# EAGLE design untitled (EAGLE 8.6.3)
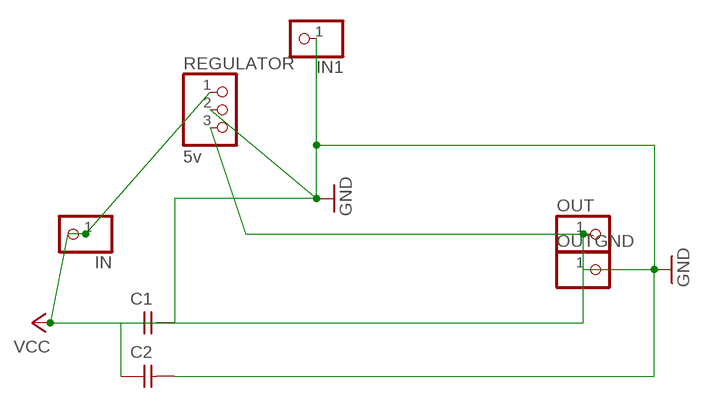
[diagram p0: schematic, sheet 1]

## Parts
C1  CAP-UNPOLARIZEDFAB  [C1206FAB]
C2  CAP-UNPOLARIZEDFAB  [C1206FAB]
IN  PINHD-1X1  [1X01]
IN1  PINHD-1X1  [1X01]
OUT  PINHD-1X1  [1X01]
OUTGND  PINHD-1X1  [1X01]
REGULATOR  5v  PINHD-1X3  [1X03]

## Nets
N$3: C2.1 OUT.1 REGULATOR.3
VCC: C1.1 IN.1 REGULATOR.1
VOLTAGEREGULATOR: C1.2 C2.2 IN1.1 OUTGND.1 REGULATOR.2 ; supply symbol labelled GND

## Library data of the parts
C1 C2 = fab:CAP-UNPOLARIZED
IN IN1 OUT OUTGND = adafruit:PINHD-1X1: Pin header 1x1 for 0.1" spacing
REGULATOR = pinhead:PINHD-1X3: PIN HEADER

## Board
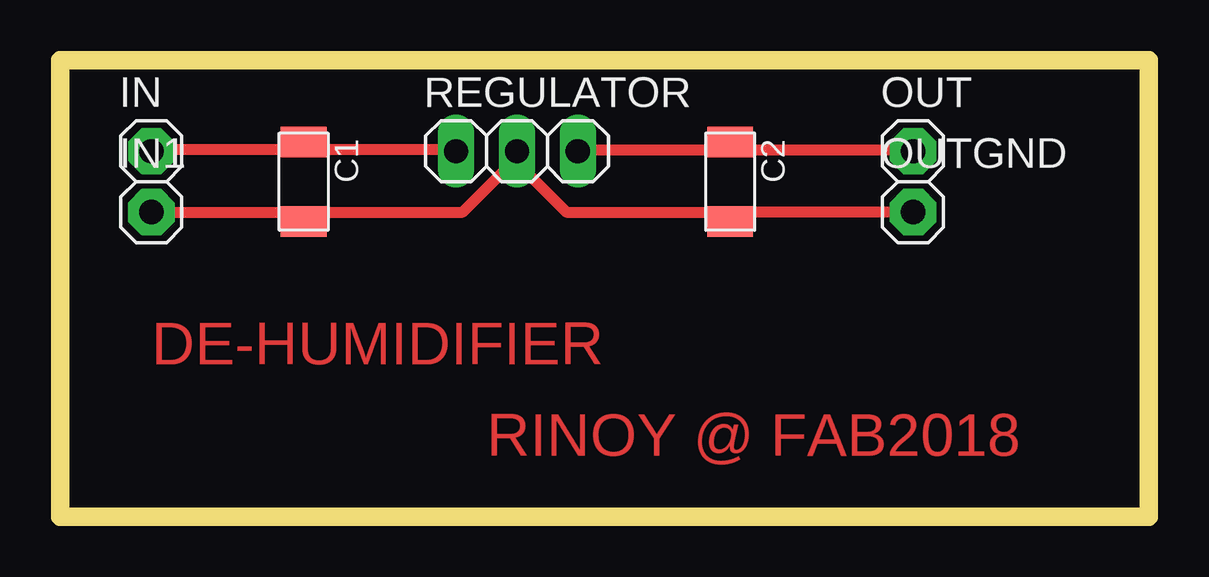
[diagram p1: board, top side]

Size 45.39 x 19.04 mm. Coordinates in mm from the lower left corner, seen from the top.
Outline: 0,0 45.39,0 45.39,19.04 0,19.04 0,0
Copper layers (1*16): Top 0.035mm / dielectric 1.5mm / Bottom 0.035mm
Design rules "default *": minimum track width 18mil, minimum drill 0.35mm, track to track 16mil, track to pad 16mil, pad to pad 16mil, via to via 16mil, smd to smd 16mil, copper to edge 40mil, drill to drill 6mil, minimum pad ring 10mil, minimum via ring 8mil, stop-mask expansion 4mil, vias tented up to drill 0mil, thermal gap 10mil

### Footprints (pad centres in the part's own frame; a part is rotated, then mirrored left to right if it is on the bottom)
C1206FAB = smd 1.27 x 1.905: 1 -1.651,0; 2 1.651,0
1X01 = drill 1.016 pad 1.93 octagon: 1 0,0
1X03 = drill 1.016 long: 1 -2.54,0; 2 0,0; 3 2.54,0

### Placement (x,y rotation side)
C1  10.16,13.97 270 top
C2  27.94,13.97 270 top
IN  3.81,15.24 0 top
IN1  3.81,12.7 0 top
OUT  35.56,15.24 0 top
OUTGND  35.56,12.7 0 top
REGULATOR  19.05,15.24 0 top

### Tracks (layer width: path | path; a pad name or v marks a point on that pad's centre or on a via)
N$3
  Top 0.457: REGULATOR.3 21.97,15.29 27.58,15.29 C2.1 28.02,15.29 35.36,15.29 OUT.1
VCC
  Top 0.457: REGULATOR.1 16.36,15.29 10.31,15.29 C1.1 9.88,15.29 3.84,15.29 IN.1
VOLTAGEREGULATOR
  Top 0.457: OUTGND.1 28.02,12.7 C2.2 27.58,12.7 21.11,12.7 18.95,14.86 | IN1.1 9.88,12.7 C1.2 10.31,12.7 16.79,12.7 18.95,14.86 | 18.95,14.86 REGULATOR.2

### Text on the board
Top: DE-HUMIDIFIER | RINOY @ FAB2018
